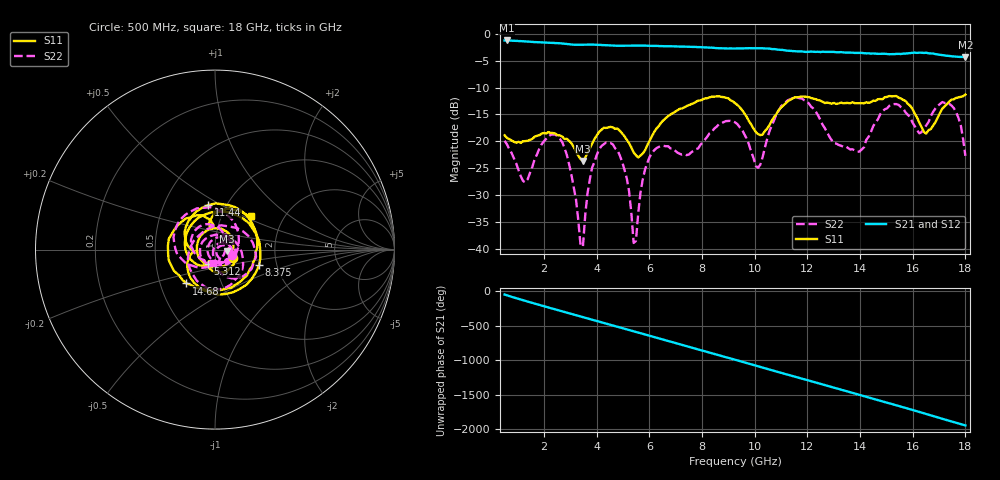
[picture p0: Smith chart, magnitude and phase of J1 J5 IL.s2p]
!Agilent Technologies,N5230A,MY45001360,A.07.50.67
!Agilent N5230A: A.07.50.67
!Date: Tuesday, April 16, 2024 17:39:37
!Correction: S11(Full 2 Port(1,2))
!S21(Full 2 Port(1,2))
!S12(Full 2 Port(1,2))
!S22(Full 2 Port(1,2))
!S2P File: Measurements: S11, S21, S12, S22:
# Hz S  dB  R 50
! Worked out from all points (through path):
!   201 points, 500 MHz to 18 GHz, reference 50 ohm
!   highest |S21| = -1.21 dB at 587.5 MHz (marker M1); lowest = -4.3 dB at 18 GHz (marker M2)
!   group delay of S21, straight-line fit = 300 ps
!   lowest |S11| = -23.6 dB at 3.475 GHz (marker M3), VSWR 1.14, Z = 57 - j0.957 ohm
!   |S11| at or under -10 dB: start of sweep to end of sweep
!   |S22| runs from -39.5 to -11.8 dB; largest |S21 - S12| = 0.0078
!   S11 on the Smith chart (normalised r, x): 500 MHz: 1.22, -0.12; 5.312 GHz: 0.91, -0.15; 8.375 GHz: 1.62, -0.30; 11.44 GHz: 0.82, +0.43; 14.68 GHz: 0.68, -0.27; 18 GHz: 1.37, +0.55
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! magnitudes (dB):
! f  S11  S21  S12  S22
! 500 MHz  -18.9  -1.2  -1.2  -19.9
! 587.5 MHz  -19.4  -1.2  -1.2  -20.6
! 1.288 GHz  -20.0  -1.4  -1.4  -27.6
! 2.6 GHz  -18.9  -1.7  -1.7  -19.6
! 3.475 GHz  -23.6  -2.0  -2.0  -39.5
! 3.825 GHz  -20.4  -2.0  -2.0  -24.9
! 4.35 GHz  -17.5  -2.1  -2.1  -20.3
! 5.312 GHz  -21.1  -2.2  -2.2  -33.3
! 5.487 GHz  -22.6  -2.2  -2.2  -38.6
! 5.838 GHz  -21.7  -2.2  -2.2  -25.2
! 6.362 GHz  -17.1  -2.3  -2.2  -21.0
! 8.375 GHz  -11.7  -2.6  -2.6  -18.2
! 9.25 GHz  -12.9  -2.7  -2.7  -16.5
! 10.12 GHz  -18.7  -2.7  -2.6  -24.9
! 11.44 GHz  -12.0  -3.2  -3.2  -12.0
! 12.22 GHz  -12.1  -3.3  -3.3  -13.9
! 13.89 GHz  -12.9  -3.5  -3.5  -21.9
! 14.68 GHz  -12.2  -3.7  -3.7  -15.9
! 15.11 GHz  -11.6  -3.8  -3.7  -13.4
! 16.51 GHz  -18.6  -3.5  -3.5  -17.1
! 17.39 GHz  -12.6  -4.1  -4.1  -13.0
! 18 GHz  -11.3  -4.3  -4.3  -22.7
